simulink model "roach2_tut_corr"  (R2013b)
settings: Solver=VariableStepDiscrete  SolverMode=SingleTasking  StartTime=0.0  StopTime=100  RelTol=1e-3
undefined symbols (not defined in the file): add_latency, addr_width, Bit, bitfield, BitWidth, bram_latency, burst_size, casper_library_scopes, conv_latency, data_width, DelayLen, fan_latency, FFTSize, FFTStage, getfield, increment, led, Location, Lower, mult_latency, mux_latency, n_bits, n_bits_data, n_inputs, n_streams, n_taps, neg_latency, negate_latency, nsamples, pfb_size, pulse_len, reset_period, ROACH, ROACH2, snapshot, sx475t, sync_period, sync_period_bits, Upper, UseCounter, Width
libraries: xbsIndex_r4 x24444, casper_library_misc x73, xbsReplacements_r4 x34, casper_library_delays x14, xps_library x7
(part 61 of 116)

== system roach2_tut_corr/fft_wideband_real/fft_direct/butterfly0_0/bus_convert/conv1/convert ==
  note: (ones_bit & 1) -> round-to-even (ones_bit ^ 1) -> round-to-odd (sign_bit & 1)-> round-to-zero (sign_bit ^ 1) -> round-to-inf (X ~| 1) -> round half down (X | 1) -> round half up
  in : Inport
  Concat : xbsIndex_r4/Concat  num_inputs=2  dbl_ovrd=off  block_type=concat
  Constant : xbsIndex_r4/Constant  const=1  gui_display_data_type=Fixed-point  arith_type=Unsigned  n_bits=1  bin_pt=0  preci_type=Single  exp_width=8  frac_width=24  explicit_period=off  period=1  equ=P=C  opselect=C  inp2=PCIN>>17  opr=+  inp1=P  carry=CIN  dbl_ovrd=off  block_type=constant
  Reinterpret : xbsIndex_r4/Reinterpret  force_arith_type=on  arith_type=Unsigned  force_bin_pt=on  bin_pt=0  block_type=reinterpret
  adder : xbsIndex_r4/AddSub  mode=Addition  use_carryin=off  use_carryout=off  en=off  latency=1  precision=User Defined  arith_type="Signed  (2's comp)"  n_bits=18  bin_pt=17  quantization=Truncate  overflow=Wrap  dbl_ovrd=off  use_behavioral_HDL=off  hw_selection=Fabric  pipelined=on  use_rpm=on  block_type=addsub
  almost_half : xbsIndex_r4/Constant  const=1  gui_display_data_type=Fixed-point  arith_type=Unsigned  n_bits=19  bin_pt=0  preci_type=Single  exp_width=8  frac_width=24  explicit_period=off  period=1  equ=P=C  opselect=C  inp2=PCIN>>17  opr=+  inp1=P  carry=CIN  dbl_ovrd=off  block_type=constant
  bit : xbsIndex_r4/Slice  nbits=1  boolean_output=off  mode=Lower Bit Location + Width  bit1=0  base1=MSB of Input  bit0=1  base0=LSB of Input  dbl_ovrd=off  block_type=slice
  force1 : xbsIndex_r4/Reinterpret  force_arith_type=on  arith_type="Signed  (2's comp)"  force_bin_pt=on  bin_pt=19  block_type=reinterpret
  force2 : xbsIndex_r4/Reinterpret  force_arith_type=off  arith_type="Signed  (2's comp)"  force_bin_pt=on  bin_pt=19  block_type=reinterpret
  tweak_op : xbsIndex_r4/Logical  logical_function=AND  inputs=2  en=off  latency=0  precision=Full  arith_type=Unsigned  n_bits=8  bin_pt=2  align_bp=on  dbl_ovrd=off  block_type=logical
  out : Outport
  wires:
  tweak_op/1 -> Concat/2
  Constant/1 -> tweak_op/2
  bit/1 -> tweak_op/1
  almost_half/1 -> force2/1
  in/1 -> Reinterpret/1, bit/1
  Concat/1 -> force1/1
  Reinterpret/1 -> Concat/1
  force1/1 -> adder/1
  force2/1 -> adder/2
  adder/1 -> out/1

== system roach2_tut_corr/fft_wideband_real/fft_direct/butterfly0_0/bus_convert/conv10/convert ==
  note: (ones_bit & 1) -> round-to-even (ones_bit ^ 1) -> round-to-odd (sign_bit & 1)-> round-to-zero (sign_bit ^ 1) -> round-to-inf (X ~| 1) -> round half down (X | 1) -> round half up
  in : Inport
  Concat : xbsIndex_r4/Concat  num_inputs=2  dbl_ovrd=off  block_type=concat
  Constant : xbsIndex_r4/Constant  const=1  gui_display_data_type=Fixed-point  arith_type=Unsigned  n_bits=1  bin_pt=0  preci_type=Single  exp_width=8  frac_width=24  explicit_period=off  period=1  equ=P=C  opselect=C  inp2=PCIN>>17  opr=+  inp1=P  carry=CIN  dbl_ovrd=off  block_type=constant
  Reinterpret : xbsIndex_r4/Reinterpret  force_arith_type=on  arith_type=Unsigned  force_bin_pt=on  bin_pt=0  block_type=reinterpret
  adder : xbsIndex_r4/AddSub  mode=Addition  use_carryin=off  use_carryout=off  en=off  latency=1  precision=User Defined  arith_type="Signed  (2's comp)"  n_bits=18  bin_pt=17  quantization=Truncate  overflow=Wrap  dbl_ovrd=off  use_behavioral_HDL=off  hw_selection=Fabric  pipelined=on  use_rpm=on  block_type=addsub
  almost_half : xbsIndex_r4/Constant  const=1  gui_display_data_type=Fixed-point  arith_type=Unsigned  n_bits=19  bin_pt=0  preci_type=Single  exp_width=8  frac_width=24  explicit_period=off  period=1  equ=P=C  opselect=C  inp2=PCIN>>17  opr=+  inp1=P  carry=CIN  dbl_ovrd=off  block_type=constant
  bit : xbsIndex_r4/Slice  nbits=1  boolean_output=off  mode=Lower Bit Location + Width  bit1=0  base1=MSB of Input  bit0=1  base0=LSB of Input  dbl_ovrd=off  block_type=slice
  force1 : xbsIndex_r4/Reinterpret  force_arith_type=on  arith_type="Signed  (2's comp)"  force_bin_pt=on  bin_pt=19  block_type=reinterpret
  force2 : xbsIndex_r4/Reinterpret  force_arith_type=off  arith_type="Signed  (2's comp)"  force_bin_pt=on  bin_pt=19  block_type=reinterpret
  tweak_op : xbsIndex_r4/Logical  logical_function=AND  inputs=2  en=off  latency=0  precision=Full  arith_type=Unsigned  n_bits=8  bin_pt=2  align_bp=on  dbl_ovrd=off  block_type=logical
  out : Outport
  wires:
  tweak_op/1 -> Concat/2
  Constant/1 -> tweak_op/2
  bit/1 -> tweak_op/1
  almost_half/1 -> force2/1
  in/1 -> Reinterpret/1, bit/1
  Concat/1 -> force1/1
  Reinterpret/1 -> Concat/1
  force1/1 -> adder/1
  force2/1 -> adder/2
  adder/1 -> out/1

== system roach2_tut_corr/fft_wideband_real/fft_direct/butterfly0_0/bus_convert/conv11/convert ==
  note: (ones_bit & 1) -> round-to-even (ones_bit ^ 1) -> round-to-odd (sign_bit & 1)-> round-to-zero (sign_bit ^ 1) -> round-to-inf (X ~| 1) -> round half down (X | 1) -> round half up
  in : Inport
  Concat : xbsIndex_r4/Concat  num_inputs=2  dbl_ovrd=off  block_type=concat
  Constant : xbsIndex_r4/Constant  const=1  gui_display_data_type=Fixed-point  arith_type=Unsigned  n_bits=1  bin_pt=0  preci_type=Single  exp_width=8  frac_width=24  explicit_period=off  period=1  equ=P=C  opselect=C  inp2=PCIN>>17  opr=+  inp1=P  carry=CIN  dbl_ovrd=off  block_type=constant
  Reinterpret : xbsIndex_r4/Reinterpret  force_arith_type=on  arith_type=Unsigned  force_bin_pt=on  bin_pt=0  block_type=reinterpret
  adder : xbsIndex_r4/AddSub  mode=Addition  use_carryin=off  use_carryout=off  en=off  latency=1  precision=User Defined  arith_type="Signed  (2's comp)"  n_bits=18  bin_pt=17  quantization=Truncate  overflow=Wrap  dbl_ovrd=off  use_behavioral_HDL=off  hw_selection=Fabric  pipelined=on  use_rpm=on  block_type=addsub
  almost_half : xbsIndex_r4/Constant  const=1  gui_display_data_type=Fixed-point  arith_type=Unsigned  n_bits=19  bin_pt=0  preci_type=Single  exp_width=8  frac_width=24  explicit_period=off  period=1  equ=P=C  opselect=C  inp2=PCIN>>17  opr=+  inp1=P  carry=CIN  dbl_ovrd=off  block_type=constant
  bit : xbsIndex_r4/Slice  nbits=1  boolean_output=off  mode=Lower Bit Location + Width  bit1=0  base1=MSB of Input  bit0=1  base0=LSB of Input  dbl_ovrd=off  block_type=slice
  force1 : xbsIndex_r4/Reinterpret  force_arith_type=on  arith_type="Signed  (2's comp)"  force_bin_pt=on  bin_pt=19  block_type=reinterpret
  force2 : xbsIndex_r4/Reinterpret  force_arith_type=off  arith_type="Signed  (2's comp)"  force_bin_pt=on  bin_pt=19  block_type=reinterpret
  tweak_op : xbsIndex_r4/Logical  logical_function=AND  inputs=2  en=off  latency=0  precision=Full  arith_type=Unsigned  n_bits=8  bin_pt=2  align_bp=on  dbl_ovrd=off  block_type=logical
  out : Outport
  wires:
  tweak_op/1 -> Concat/2
  Constant/1 -> tweak_op/2
  bit/1 -> tweak_op/1
  almost_half/1 -> force2/1
  in/1 -> Reinterpret/1, bit/1
  Concat/1 -> force1/1
  Reinterpret/1 -> Concat/1
  force1/1 -> adder/1
  force2/1 -> adder/2
  adder/1 -> out/1

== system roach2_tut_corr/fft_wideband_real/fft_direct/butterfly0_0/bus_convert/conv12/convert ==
  note: (ones_bit & 1) -> round-to-even (ones_bit ^ 1) -> round-to-odd (sign_bit & 1)-> round-to-zero (sign_bit ^ 1) -> round-to-inf (X ~| 1) -> round half down (X | 1) -> round half up
  in : Inport
  Concat : xbsIndex_r4/Concat  num_inputs=2  dbl_ovrd=off  block_type=concat
  Constant : xbsIndex_r4/Constant  const=1  gui_display_data_type=Fixed-point  arith_type=Unsigned  n_bits=1  bin_pt=0  preci_type=Single  exp_width=8  frac_width=24  explicit_period=off  period=1  equ=P=C  opselect=C  inp2=PCIN>>17  opr=+  inp1=P  carry=CIN  dbl_ovrd=off  block_type=constant
  Reinterpret : xbsIndex_r4/Reinterpret  force_arith_type=on  arith_type=Unsigned  force_bin_pt=on  bin_pt=0  block_type=reinterpret
  adder : xbsIndex_r4/AddSub  mode=Addition  use_carryin=off  use_carryout=off  en=off  latency=1  precision=User Defined  arith_type="Signed  (2's comp)"  n_bits=18  bin_pt=17  quantization=Truncate  overflow=Wrap  dbl_ovrd=off  use_behavioral_HDL=off  hw_selection=Fabric  pipelined=on  use_rpm=on  block_type=addsub
  almost_half : xbsIndex_r4/Constant  const=1  gui_display_data_type=Fixed-point  arith_type=Unsigned  n_bits=19  bin_pt=0  preci_type=Single  exp_width=8  frac_width=24  explicit_period=off  period=1  equ=P=C  opselect=C  inp2=PCIN>>17  opr=+  inp1=P  carry=CIN  dbl_ovrd=off  block_type=constant
  bit : xbsIndex_r4/Slice  nbits=1  boolean_output=off  mode=Lower Bit Location + Width  bit1=0  base1=MSB of Input  bit0=1  base0=LSB of Input  dbl_ovrd=off  block_type=slice
  force1 : xbsIndex_r4/Reinterpret  force_arith_type=on  arith_type="Signed  (2's comp)"  force_bin_pt=on  bin_pt=19  block_type=reinterpret
  force2 : xbsIndex_r4/Reinterpret  force_arith_type=off  arith_type="Signed  (2's comp)"  force_bin_pt=on  bin_pt=19  block_type=reinterpret
  tweak_op : xbsIndex_r4/Logical  logical_function=AND  inputs=2  en=off  latency=0  precision=Full  arith_type=Unsigned  n_bits=8  bin_pt=2  align_bp=on  dbl_ovrd=off  block_type=logical
  out : Outport
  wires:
  tweak_op/1 -> Concat/2
  Constant/1 -> tweak_op/2
  bit/1 -> tweak_op/1
  almost_half/1 -> force2/1
  in/1 -> Reinterpret/1, bit/1
  Concat/1 -> force1/1
  Reinterpret/1 -> Concat/1
  force1/1 -> adder/1
  force2/1 -> adder/2
  adder/1 -> out/1

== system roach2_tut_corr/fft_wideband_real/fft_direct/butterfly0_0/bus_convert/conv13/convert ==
  note: (ones_bit & 1) -> round-to-even (ones_bit ^ 1) -> round-to-odd (sign_bit & 1)-> round-to-zero (sign_bit ^ 1) -> round-to-inf (X ~| 1) -> round half down (X | 1) -> round half up
  in : Inport
  Concat : xbsIndex_r4/Concat  num_inputs=2  dbl_ovrd=off  block_type=concat
  Constant : xbsIndex_r4/Constant  const=1  gui_display_data_type=Fixed-point  arith_type=Unsigned  n_bits=1  bin_pt=0  preci_type=Single  exp_width=8  frac_width=24  explicit_period=off  period=1  equ=P=C  opselect=C  inp2=PCIN>>17  opr=+  inp1=P  carry=CIN  dbl_ovrd=off  block_type=constant
  Reinterpret : xbsIndex_r4/Reinterpret  force_arith_type=on  arith_type=Unsigned  force_bin_pt=on  bin_pt=0  block_type=reinterpret
  adder : xbsIndex_r4/AddSub  mode=Addition  use_carryin=off  use_carryout=off  en=off  latency=1  precision=User Defined  arith_type="Signed  (2's comp)"  n_bits=18  bin_pt=17  quantization=Truncate  overflow=Wrap  dbl_ovrd=off  use_behavioral_HDL=off  hw_selection=Fabric  pipelined=on  use_rpm=on  block_type=addsub
  almost_half : xbsIndex_r4/Constant  const=1  gui_display_data_type=Fixed-point  arith_type=Unsigned  n_bits=19  bin_pt=0  preci_type=Single  exp_width=8  frac_width=24  explicit_period=off  period=1  equ=P=C  opselect=C  inp2=PCIN>>17  opr=+  inp1=P  carry=CIN  dbl_ovrd=off  block_type=constant
  bit : xbsIndex_r4/Slice  nbits=1  boolean_output=off  mode=Lower Bit Location + Width  bit1=0  base1=MSB of Input  bit0=1  base0=LSB of Input  dbl_ovrd=off  block_type=slice
  force1 : xbsIndex_r4/Reinterpret  force_arith_type=on  arith_type="Signed  (2's comp)"  force_bin_pt=on  bin_pt=19  block_type=reinterpret
  force2 : xbsIndex_r4/Reinterpret  force_arith_type=off  arith_type="Signed  (2's comp)"  force_bin_pt=on  bin_pt=19  block_type=reinterpret
  tweak_op : xbsIndex_r4/Logical  logical_function=AND  inputs=2  en=off  latency=0  precision=Full  arith_type=Unsigned  n_bits=8  bin_pt=2  align_bp=on  dbl_ovrd=off  block_type=logical
  out : Outport
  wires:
  tweak_op/1 -> Concat/2
  Constant/1 -> tweak_op/2
  bit/1 -> tweak_op/1
  almost_half/1 -> force2/1
  in/1 -> Reinterpret/1, bit/1
  Concat/1 -> force1/1
  Reinterpret/1 -> Concat/1
  force1/1 -> adder/1
  force2/1 -> adder/2
  adder/1 -> out/1

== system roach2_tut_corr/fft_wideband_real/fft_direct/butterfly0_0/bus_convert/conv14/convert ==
  note: (ones_bit & 1) -> round-to-even (ones_bit ^ 1) -> round-to-odd (sign_bit & 1)-> round-to-zero (sign_bit ^ 1) -> round-to-inf (X ~| 1) -> round half down (X | 1) -> round half up
  in : Inport
  Concat : xbsIndex_r4/Concat  num_inputs=2  dbl_ovrd=off  block_type=concat
  Constant : xbsIndex_r4/Constant  const=1  gui_display_data_type=Fixed-point  arith_type=Unsigned  n_bits=1  bin_pt=0  preci_type=Single  exp_width=8  frac_width=24  explicit_period=off  period=1  equ=P=C  opselect=C  inp2=PCIN>>17  opr=+  inp1=P  carry=CIN  dbl_ovrd=off  block_type=constant
  Reinterpret : xbsIndex_r4/Reinterpret  force_arith_type=on  arith_type=Unsigned  force_bin_pt=on  bin_pt=0  block_type=reinterpret
  adder : xbsIndex_r4/AddSub  mode=Addition  use_carryin=off  use_carryout=off  en=off  latency=1  precision=User Defined  arith_type="Signed  (2's comp)"  n_bits=18  bin_pt=17  quantization=Truncate  overflow=Wrap  dbl_ovrd=off  use_behavioral_HDL=off  hw_selection=Fabric  pipelined=on  use_rpm=on  block_type=addsub
  almost_half : xbsIndex_r4/Constant  const=1  gui_display_data_type=Fixed-point  arith_type=Unsigned  n_bits=19  bin_pt=0  preci_type=Single  exp_width=8  frac_width=24  explicit_period=off  period=1  equ=P=C  opselect=C  inp2=PCIN>>17  opr=+  inp1=P  carry=CIN  dbl_ovrd=off  block_type=constant
  bit : xbsIndex_r4/Slice  nbits=1  boolean_output=off  mode=Lower Bit Location + Width  bit1=0  base1=MSB of Input  bit0=1  base0=LSB of Input  dbl_ovrd=off  block_type=slice
  force1 : xbsIndex_r4/Reinterpret  force_arith_type=on  arith_type="Signed  (2's comp)"  force_bin_pt=on  bin_pt=19  block_type=reinterpret
  force2 : xbsIndex_r4/Reinterpret  force_arith_type=off  arith_type="Signed  (2's comp)"  force_bin_pt=on  bin_pt=19  block_type=reinterpret
  tweak_op : xbsIndex_r4/Logical  logical_function=AND  inputs=2  en=off  latency=0  precision=Full  arith_type=Unsigned  n_bits=8  bin_pt=2  align_bp=on  dbl_ovrd=off  block_type=logical
  out : Outport
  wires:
  tweak_op/1 -> Concat/2
  Constant/1 -> tweak_op/2
  bit/1 -> tweak_op/1
  almost_half/1 -> force2/1
  in/1 -> Reinterpret/1, bit/1
  Concat/1 -> force1/1
  Reinterpret/1 -> Concat/1
  force1/1 -> adder/1
  force2/1 -> adder/2
  adder/1 -> out/1

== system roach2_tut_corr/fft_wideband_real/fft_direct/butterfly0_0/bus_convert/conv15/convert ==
  note: (ones_bit & 1) -> round-to-even (ones_bit ^ 1) -> round-to-odd (sign_bit & 1)-> round-to-zero (sign_bit ^ 1) -> round-to-inf (X ~| 1) -> round half down (X | 1) -> round half up
  in : Inport
  Concat : xbsIndex_r4/Concat  num_inputs=2  dbl_ovrd=off  block_type=concat
  Constant : xbsIndex_r4/Constant  const=1  gui_display_data_type=Fixed-point  arith_type=Unsigned  n_bits=1  bin_pt=0  preci_type=Single  exp_width=8  frac_width=24  explicit_period=off  period=1  equ=P=C  opselect=C  inp2=PCIN>>17  opr=+  inp1=P  carry=CIN  dbl_ovrd=off  block_type=constant
  Reinterpret : xbsIndex_r4/Reinterpret  force_arith_type=on  arith_type=Unsigned  force_bin_pt=on  bin_pt=0  block_type=reinterpret
  adder : xbsIndex_r4/AddSub  mode=Addition  use_carryin=off  use_carryout=off  en=off  latency=1  precision=User Defined  arith_type="Signed  (2's comp)"  n_bits=18  bin_pt=17  quantization=Truncate  overflow=Wrap  dbl_ovrd=off  use_behavioral_HDL=off  hw_selection=Fabric  pipelined=on  use_rpm=on  block_type=addsub
  almost_half : xbsIndex_r4/Constant  const=1  gui_display_data_type=Fixed-point  arith_type=Unsigned  n_bits=19  bin_pt=0  preci_type=Single  exp_width=8  frac_width=24  explicit_period=off  period=1  equ=P=C  opselect=C  inp2=PCIN>>17  opr=+  inp1=P  carry=CIN  dbl_ovrd=off  block_type=constant
  bit : xbsIndex_r4/Slice  nbits=1  boolean_output=off  mode=Lower Bit Location + Width  bit1=0  base1=MSB of Input  bit0=1  base0=LSB of Input  dbl_ovrd=off  block_type=slice
  force1 : xbsIndex_r4/Reinterpret  force_arith_type=on  arith_type="Signed  (2's comp)"  force_bin_pt=on  bin_pt=19  block_type=reinterpret
  force2 : xbsIndex_r4/Reinterpret  force_arith_type=off  arith_type="Signed  (2's comp)"  force_bin_pt=on  bin_pt=19  block_type=reinterpret
  tweak_op : xbsIndex_r4/Logical  logical_function=AND  inputs=2  en=off  latency=0  precision=Full  arith_type=Unsigned  n_bits=8  bin_pt=2  align_bp=on  dbl_ovrd=off  block_type=logical
  out : Outport
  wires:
  tweak_op/1 -> Concat/2
  Constant/1 -> tweak_op/2
  bit/1 -> tweak_op/1
  almost_half/1 -> force2/1
  in/1 -> Reinterpret/1, bit/1
  Concat/1 -> force1/1
  Reinterpret/1 -> Concat/1
  force1/1 -> adder/1
  force2/1 -> adder/2
  adder/1 -> out/1

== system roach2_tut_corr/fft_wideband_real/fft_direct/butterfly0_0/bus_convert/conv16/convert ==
  note: (ones_bit & 1) -> round-to-even (ones_bit ^ 1) -> round-to-odd (sign_bit & 1)-> round-to-zero (sign_bit ^ 1) -> round-to-inf (X ~| 1) -> round half down (X | 1) -> round half up
  in : Inport
  Concat : xbsIndex_r4/Concat  num_inputs=2  dbl_ovrd=off  block_type=concat
  Constant : xbsIndex_r4/Constant  const=1  gui_display_data_type=Fixed-point  arith_type=Unsigned  n_bits=1  bin_pt=0  preci_type=Single  exp_width=8  frac_width=24  explicit_period=off  period=1  equ=P=C  opselect=C  inp2=PCIN>>17  opr=+  inp1=P  carry=CIN  dbl_ovrd=off  block_type=constant
  Reinterpret : xbsIndex_r4/Reinterpret  force_arith_type=on  arith_type=Unsigned  force_bin_pt=on  bin_pt=0  block_type=reinterpret
  adder : xbsIndex_r4/AddSub  mode=Addition  use_carryin=off  use_carryout=off  en=off  latency=1  precision=User Defined  arith_type="Signed  (2's comp)"  n_bits=18  bin_pt=17  quantization=Truncate  overflow=Wrap  dbl_ovrd=off  use_behavioral_HDL=off  hw_selection=Fabric  pipelined=on  use_rpm=on  block_type=addsub
  almost_half : xbsIndex_r4/Constant  const=1  gui_display_data_type=Fixed-point  arith_type=Unsigned  n_bits=19  bin_pt=0  preci_type=Single  exp_width=8  frac_width=24  explicit_period=off  period=1  equ=P=C  opselect=C  inp2=PCIN>>17  opr=+  inp1=P  carry=CIN  dbl_ovrd=off  block_type=constant
  bit : xbsIndex_r4/Slice  nbits=1  boolean_output=off  mode=Lower Bit Location + Width  bit1=0  base1=MSB of Input  bit0=1  base0=LSB of Input  dbl_ovrd=off  block_type=slice
  force1 : xbsIndex_r4/Reinterpret  force_arith_type=on  arith_type="Signed  (2's comp)"  force_bin_pt=on  bin_pt=19  block_type=reinterpret
  force2 : xbsIndex_r4/Reinterpret  force_arith_type=off  arith_type="Signed  (2's comp)"  force_bin_pt=on  bin_pt=19  block_type=reinterpret
  tweak_op : xbsIndex_r4/Logical  logical_function=AND  inputs=2  en=off  latency=0  precision=Full  arith_type=Unsigned  n_bits=8  bin_pt=2  align_bp=on  dbl_ovrd=off  block_type=logical
  out : Outport
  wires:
  tweak_op/1 -> Concat/2
  Constant/1 -> tweak_op/2
  bit/1 -> tweak_op/1
  almost_half/1 -> force2/1
  in/1 -> Reinterpret/1, bit/1
  Concat/1 -> force1/1
  Reinterpret/1 -> Concat/1
  force1/1 -> adder/1
  force2/1 -> adder/2
  adder/1 -> out/1

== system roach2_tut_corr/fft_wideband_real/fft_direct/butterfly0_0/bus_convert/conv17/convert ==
  note: (ones_bit & 1) -> round-to-even (ones_bit ^ 1) -> round-to-odd (sign_bit & 1)-> round-to-zero (sign_bit ^ 1) -> round-to-inf (X ~| 1) -> round half down (X | 1) -> round half up
  in : Inport
  Concat : xbsIndex_r4/Concat  num_inputs=2  dbl_ovrd=off  block_type=concat
  Constant : xbsIndex_r4/Constant  const=1  gui_display_data_type=Fixed-point  arith_type=Unsigned  n_bits=1  bin_pt=0  preci_type=Single  exp_width=8  frac_width=24  explicit_period=off  period=1  equ=P=C  opselect=C  inp2=PCIN>>17  opr=+  inp1=P  carry=CIN  dbl_ovrd=off  block_type=constant
  Reinterpret : xbsIndex_r4/Reinterpret  force_arith_type=on  arith_type=Unsigned  force_bin_pt=on  bin_pt=0  block_type=reinterpret
  adder : xbsIndex_r4/AddSub  mode=Addition  use_carryin=off  use_carryout=off  en=off  latency=1  precision=User Defined  arith_type="Signed  (2's comp)"  n_bits=18  bin_pt=17  quantization=Truncate  overflow=Wrap  dbl_ovrd=off  use_behavioral_HDL=off  hw_selection=Fabric  pipelined=on  use_rpm=on  block_type=addsub
  almost_half : xbsIndex_r4/Constant  const=1  gui_display_data_type=Fixed-point  arith_type=Unsigned  n_bits=19  bin_pt=0  preci_type=Single  exp_width=8  frac_width=24  explicit_period=off  period=1  equ=P=C  opselect=C  inp2=PCIN>>17  opr=+  inp1=P  carry=CIN  dbl_ovrd=off  block_type=constant
  bit : xbsIndex_r4/Slice  nbits=1  boolean_output=off  mode=Lower Bit Location + Width  bit1=0  base1=MSB of Input  bit0=1  base0=LSB of Input  dbl_ovrd=off  block_type=slice
  force1 : xbsIndex_r4/Reinterpret  force_arith_type=on  arith_type="Signed  (2's comp)"  force_bin_pt=on  bin_pt=19  block_type=reinterpret
  force2 : xbsIndex_r4/Reinterpret  force_arith_type=off  arith_type="Signed  (2's comp)"  force_bin_pt=on  bin_pt=19  block_type=reinterpret
  tweak_op : xbsIndex_r4/Logical  logical_function=AND  inputs=2  en=off  latency=0  precision=Full  arith_type=Unsigned  n_bits=8  bin_pt=2  align_bp=on  dbl_ovrd=off  block_type=logical
  out : Outport
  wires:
  tweak_op/1 -> Concat/2
  Constant/1 -> tweak_op/2
  bit/1 -> tweak_op/1
  almost_half/1 -> force2/1
  in/1 -> Reinterpret/1, bit/1
  Concat/1 -> force1/1
  Reinterpret/1 -> Concat/1
  force1/1 -> adder/1
  force2/1 -> adder/2
  adder/1 -> out/1

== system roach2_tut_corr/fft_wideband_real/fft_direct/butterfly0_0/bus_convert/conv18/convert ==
  note: (ones_bit & 1) -> round-to-even (ones_bit ^ 1) -> round-to-odd (sign_bit & 1)-> round-to-zero (sign_bit ^ 1) -> round-to-inf (X ~| 1) -> round half down (X | 1) -> round half up
  in : Inport
  Concat : xbsIndex_r4/Concat  num_inputs=2  dbl_ovrd=off  block_type=concat
  Constant : xbsIndex_r4/Constant  const=1  gui_display_data_type=Fixed-point  arith_type=Unsigned  n_bits=1  bin_pt=0  preci_type=Single  exp_width=8  frac_width=24  explicit_period=off  period=1  equ=P=C  opselect=C  inp2=PCIN>>17  opr=+  inp1=P  carry=CIN  dbl_ovrd=off  block_type=constant
  Reinterpret : xbsIndex_r4/Reinterpret  force_arith_type=on  arith_type=Unsigned  force_bin_pt=on  bin_pt=0  block_type=reinterpret
  adder : xbsIndex_r4/AddSub  mode=Addition  use_carryin=off  use_carryout=off  en=off  latency=1  precision=User Defined  arith_type="Signed  (2's comp)"  n_bits=18  bin_pt=17  quantization=Truncate  overflow=Wrap  dbl_ovrd=off  use_behavioral_HDL=off  hw_selection=Fabric  pipelined=on  use_rpm=on  block_type=addsub
  almost_half : xbsIndex_r4/Constant  const=1  gui_display_data_type=Fixed-point  arith_type=Unsigned  n_bits=19  bin_pt=0  preci_type=Single  exp_width=8  frac_width=24  explicit_period=off  period=1  equ=P=C  opselect=C  inp2=PCIN>>17  opr=+  inp1=P  carry=CIN  dbl_ovrd=off  block_type=constant
  bit : xbsIndex_r4/Slice  nbits=1  boolean_output=off  mode=Lower Bit Location + Width  bit1=0  base1=MSB of Input  bit0=1  base0=LSB of Input  dbl_ovrd=off  block_type=slice
  force1 : xbsIndex_r4/Reinterpret  force_arith_type=on  arith_type="Signed  (2's comp)"  force_bin_pt=on  bin_pt=19  block_type=reinterpret
  force2 : xbsIndex_r4/Reinterpret  force_arith_type=off  arith_type="Signed  (2's comp)"  force_bin_pt=on  bin_pt=19  block_type=reinterpret
  tweak_op : xbsIndex_r4/Logical  logical_function=AND  inputs=2  en=off  latency=0  precision=Full  arith_type=Unsigned  n_bits=8  bin_pt=2  align_bp=on  dbl_ovrd=off  block_type=logical
  out : Outport
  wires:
  tweak_op/1 -> Concat/2
  Constant/1 -> tweak_op/2
  bit/1 -> tweak_op/1
  almost_half/1 -> force2/1
  in/1 -> Reinterpret/1, bit/1
  Concat/1 -> force1/1
  Reinterpret/1 -> Concat/1
  force1/1 -> adder/1
  force2/1 -> adder/2
  adder/1 -> out/1

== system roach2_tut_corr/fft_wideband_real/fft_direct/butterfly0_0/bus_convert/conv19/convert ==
  note: (ones_bit & 1) -> round-to-even (ones_bit ^ 1) -> round-to-odd (sign_bit & 1)-> round-to-zero (sign_bit ^ 1) -> round-to-inf (X ~| 1) -> round half down (X | 1) -> round half up
  in : Inport
  Concat : xbsIndex_r4/Concat  num_inputs=2  dbl_ovrd=off  block_type=concat
  Constant : xbsIndex_r4/Constant  const=1  gui_display_data_type=Fixed-point  arith_type=Unsigned  n_bits=1  bin_pt=0  preci_type=Single  exp_width=8  frac_width=24  explicit_period=off  period=1  equ=P=C  opselect=C  inp2=PCIN>>17  opr=+  inp1=P  carry=CIN  dbl_ovrd=off  block_type=constant
  Reinterpret : xbsIndex_r4/Reinterpret  force_arith_type=on  arith_type=Unsigned  force_bin_pt=on  bin_pt=0  block_type=reinterpret
  adder : xbsIndex_r4/AddSub  mode=Addition  use_carryin=off  use_carryout=off  en=off  latency=1  precision=User Defined  arith_type="Signed  (2's comp)"  n_bits=18  bin_pt=17  quantization=Truncate  overflow=Wrap  dbl_ovrd=off  use_behavioral_HDL=off  hw_selection=Fabric  pipelined=on  use_rpm=on  block_type=addsub
  almost_half : xbsIndex_r4/Constant  const=1  gui_display_data_type=Fixed-point  arith_type=Unsigned  n_bits=19  bin_pt=0  preci_type=Single  exp_width=8  frac_width=24  explicit_period=off  period=1  equ=P=C  opselect=C  inp2=PCIN>>17  opr=+  inp1=P  carry=CIN  dbl_ovrd=off  block_type=constant
  bit : xbsIndex_r4/Slice  nbits=1  boolean_output=off  mode=Lower Bit Location + Width  bit1=0  base1=MSB of Input  bit0=1  base0=LSB of Input  dbl_ovrd=off  block_type=slice
  force1 : xbsIndex_r4/Reinterpret  force_arith_type=on  arith_type="Signed  (2's comp)"  force_bin_pt=on  bin_pt=19  block_type=reinterpret
  force2 : xbsIndex_r4/Reinterpret  force_arith_type=off  arith_type="Signed  (2's comp)"  force_bin_pt=on  bin_pt=19  block_type=reinterpret
  tweak_op : xbsIndex_r4/Logical  logical_function=AND  inputs=2  en=off  latency=0  precision=Full  arith_type=Unsigned  n_bits=8  bin_pt=2  align_bp=on  dbl_ovrd=off  block_type=logical
  out : Outport
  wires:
  tweak_op/1 -> Concat/2
  Constant/1 -> tweak_op/2
  bit/1 -> tweak_op/1
  almost_half/1 -> force2/1
  in/1 -> Reinterpret/1, bit/1
  Concat/1 -> force1/1
  Reinterpret/1 -> Concat/1
  force1/1 -> adder/1
  force2/1 -> adder/2
  adder/1 -> out/1

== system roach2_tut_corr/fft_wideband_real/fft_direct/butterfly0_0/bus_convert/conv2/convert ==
  note: (ones_bit & 1) -> round-to-even (ones_bit ^ 1) -> round-to-odd (sign_bit & 1)-> round-to-zero (sign_bit ^ 1) -> round-to-inf (X ~| 1) -> round half down (X | 1) -> round half up
  in : Inport
  Concat : xbsIndex_r4/Concat  num_inputs=2  dbl_ovrd=off  block_type=concat
  Constant : xbsIndex_r4/Constant  const=1  gui_display_data_type=Fixed-point  arith_type=Unsigned  n_bits=1  bin_pt=0  preci_type=Single  exp_width=8  frac_width=24  explicit_period=off  period=1  equ=P=C  opselect=C  inp2=PCIN>>17  opr=+  inp1=P  carry=CIN  dbl_ovrd=off  block_type=constant
  Reinterpret : xbsIndex_r4/Reinterpret  force_arith_type=on  arith_type=Unsigned  force_bin_pt=on  bin_pt=0  block_type=reinterpret
  adder : xbsIndex_r4/AddSub  mode=Addition  use_carryin=off  use_carryout=off  en=off  latency=1  precision=User Defined  arith_type="Signed  (2's comp)"  n_bits=18  bin_pt=17  quantization=Truncate  overflow=Wrap  dbl_ovrd=off  use_behavioral_HDL=off  hw_selection=Fabric  pipelined=on  use_rpm=on  block_type=addsub
  almost_half : xbsIndex_r4/Constant  const=1  gui_display_data_type=Fixed-point  arith_type=Unsigned  n_bits=19  bin_pt=0  preci_type=Single  exp_width=8  frac_width=24  explicit_period=off  period=1  equ=P=C  opselect=C  inp2=PCIN>>17  opr=+  inp1=P  carry=CIN  dbl_ovrd=off  block_type=constant
  bit : xbsIndex_r4/Slice  nbits=1  boolean_output=off  mode=Lower Bit Location + Width  bit1=0  base1=MSB of Input  bit0=1  base0=LSB of Input  dbl_ovrd=off  block_type=slice
  force1 : xbsIndex_r4/Reinterpret  force_arith_type=on  arith_type="Signed  (2's comp)"  force_bin_pt=on  bin_pt=19  block_type=reinterpret
  force2 : xbsIndex_r4/Reinterpret  force_arith_type=off  arith_type="Signed  (2's comp)"  force_bin_pt=on  bin_pt=19  block_type=reinterpret
  tweak_op : xbsIndex_r4/Logical  logical_function=AND  inputs=2  en=off  latency=0  precision=Full  arith_type=Unsigned  n_bits=8  bin_pt=2  align_bp=on  dbl_ovrd=off  block_type=logical
  out : Outport
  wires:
  tweak_op/1 -> Concat/2
  Constant/1 -> tweak_op/2
  bit/1 -> tweak_op/1
  almost_half/1 -> force2/1
  in/1 -> Reinterpret/1, bit/1
  Concat/1 -> force1/1
  Reinterpret/1 -> Concat/1
  force1/1 -> adder/1
  force2/1 -> adder/2
  adder/1 -> out/1

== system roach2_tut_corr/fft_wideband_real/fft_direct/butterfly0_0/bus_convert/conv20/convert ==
  note: (ones_bit & 1) -> round-to-even (ones_bit ^ 1) -> round-to-odd (sign_bit & 1)-> round-to-zero (sign_bit ^ 1) -> round-to-inf (X ~| 1) -> round half down (X | 1) -> round half up
  in : Inport
  Concat : xbsIndex_r4/Concat  num_inputs=2  dbl_ovrd=off  block_type=concat
  Constant : xbsIndex_r4/Constant  const=1  gui_display_data_type=Fixed-point  arith_type=Unsigned  n_bits=1  bin_pt=0  preci_type=Single  exp_width=8  frac_width=24  explicit_period=off  period=1  equ=P=C  opselect=C  inp2=PCIN>>17  opr=+  inp1=P  carry=CIN  dbl_ovrd=off  block_type=constant
  Reinterpret : xbsIndex_r4/Reinterpret  force_arith_type=on  arith_type=Unsigned  force_bin_pt=on  bin_pt=0  block_type=reinterpret
  adder : xbsIndex_r4/AddSub  mode=Addition  use_carryin=off  use_carryout=off  en=off  latency=1  precision=User Defined  arith_type="Signed  (2's comp)"  n_bits=18  bin_pt=17  quantization=Truncate  overflow=Wrap  dbl_ovrd=off  use_behavioral_HDL=off  hw_selection=Fabric  pipelined=on  use_rpm=on  block_type=addsub
  almost_half : xbsIndex_r4/Constant  const=1  gui_display_data_type=Fixed-point  arith_type=Unsigned  n_bits=19  bin_pt=0  preci_type=Single  exp_width=8  frac_width=24  explicit_period=off  period=1  equ=P=C  opselect=C  inp2=PCIN>>17  opr=+  inp1=P  carry=CIN  dbl_ovrd=off  block_type=constant
  bit : xbsIndex_r4/Slice  nbits=1  boolean_output=off  mode=Lower Bit Location + Width  bit1=0  base1=MSB of Input  bit0=1  base0=LSB of Input  dbl_ovrd=off  block_type=slice
  force1 : xbsIndex_r4/Reinterpret  force_arith_type=on  arith_type="Signed  (2's comp)"  force_bin_pt=on  bin_pt=19  block_type=reinterpret
  force2 : xbsIndex_r4/Reinterpret  force_arith_type=off  arith_type="Signed  (2's comp)"  force_bin_pt=on  bin_pt=19  block_type=reinterpret
  tweak_op : xbsIndex_r4/Logical  logical_function=AND  inputs=2  en=off  latency=0  precision=Full  arith_type=Unsigned  n_bits=8  bin_pt=2  align_bp=on  dbl_ovrd=off  block_type=logical
  out : Outport
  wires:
  tweak_op/1 -> Concat/2
  Constant/1 -> tweak_op/2
  bit/1 -> tweak_op/1
  almost_half/1 -> force2/1
  in/1 -> Reinterpret/1, bit/1
  Concat/1 -> force1/1
  Reinterpret/1 -> Concat/1
  force1/1 -> adder/1
  force2/1 -> adder/2
  adder/1 -> out/1

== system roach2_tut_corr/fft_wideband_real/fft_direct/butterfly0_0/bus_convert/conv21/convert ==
  note: (ones_bit & 1) -> round-to-even (ones_bit ^ 1) -> round-to-odd (sign_bit & 1)-> round-to-zero (sign_bit ^ 1) -> round-to-inf (X ~| 1) -> round half down (X | 1) -> round half up
  in : Inport
  Concat : xbsIndex_r4/Concat  num_inputs=2  dbl_ovrd=off  block_type=concat
  Constant : xbsIndex_r4/Constant  const=1  gui_display_data_type=Fixed-point  arith_type=Unsigned  n_bits=1  bin_pt=0  preci_type=Single  exp_width=8  frac_width=24  explicit_period=off  period=1  equ=P=C  opselect=C  inp2=PCIN>>17  opr=+  inp1=P  carry=CIN  dbl_ovrd=off  block_type=constant
  Reinterpret : xbsIndex_r4/Reinterpret  force_arith_type=on  arith_type=Unsigned  force_bin_pt=on  bin_pt=0  block_type=reinterpret
  adder : xbsIndex_r4/AddSub  mode=Addition  use_carryin=off  use_carryout=off  en=off  latency=1  precision=User Defined  arith_type="Signed  (2's comp)"  n_bits=18  bin_pt=17  quantization=Truncate  overflow=Wrap  dbl_ovrd=off  use_behavioral_HDL=off  hw_selection=Fabric  pipelined=on  use_rpm=on  block_type=addsub
  almost_half : xbsIndex_r4/Constant  const=1  gui_display_data_type=Fixed-point  arith_type=Unsigned  n_bits=19  bin_pt=0  preci_type=Single  exp_width=8  frac_width=24  explicit_period=off  period=1  equ=P=C  opselect=C  inp2=PCIN>>17  opr=+  inp1=P  carry=CIN  dbl_ovrd=off  block_type=constant
  bit : xbsIndex_r4/Slice  nbits=1  boolean_output=off  mode=Lower Bit Location + Width  bit1=0  base1=MSB of Input  bit0=1  base0=LSB of Input  dbl_ovrd=off  block_type=slice
  force1 : xbsIndex_r4/Reinterpret  force_arith_type=on  arith_type="Signed  (2's comp)"  force_bin_pt=on  bin_pt=19  block_type=reinterpret
  force2 : xbsIndex_r4/Reinterpret  force_arith_type=off  arith_type="Signed  (2's comp)"  force_bin_pt=on  bin_pt=19  block_type=reinterpret
  tweak_op : xbsIndex_r4/Logical  logical_function=AND  inputs=2  en=off  latency=0  precision=Full  arith_type=Unsigned  n_bits=8  bin_pt=2  align_bp=on  dbl_ovrd=off  block_type=logical
  out : Outport
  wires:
  tweak_op/1 -> Concat/2
  Constant/1 -> tweak_op/2
  bit/1 -> tweak_op/1
  almost_half/1 -> force2/1
  in/1 -> Reinterpret/1, bit/1
  Concat/1 -> force1/1
  Reinterpret/1 -> Concat/1
  force1/1 -> adder/1
  force2/1 -> adder/2
  adder/1 -> out/1

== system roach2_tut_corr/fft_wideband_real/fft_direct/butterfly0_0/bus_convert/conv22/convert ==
  note: (ones_bit & 1) -> round-to-even (ones_bit ^ 1) -> round-to-odd (sign_bit & 1)-> round-to-zero (sign_bit ^ 1) -> round-to-inf (X ~| 1) -> round half down (X | 1) -> round half up
  in : Inport
  Concat : xbsIndex_r4/Concat  num_inputs=2  dbl_ovrd=off  block_type=concat
  Constant : xbsIndex_r4/Constant  const=1  gui_display_data_type=Fixed-point  arith_type=Unsigned  n_bits=1  bin_pt=0  preci_type=Single  exp_width=8  frac_width=24  explicit_period=off  period=1  equ=P=C  opselect=C  inp2=PCIN>>17  opr=+  inp1=P  carry=CIN  dbl_ovrd=off  block_type=constant
  Reinterpret : xbsIndex_r4/Reinterpret  force_arith_type=on  arith_type=Unsigned  force_bin_pt=on  bin_pt=0  block_type=reinterpret
  adder : xbsIndex_r4/AddSub  mode=Addition  use_carryin=off  use_carryout=off  en=off  latency=1  precision=User Defined  arith_type="Signed  (2's comp)"  n_bits=18  bin_pt=17  quantization=Truncate  overflow=Wrap  dbl_ovrd=off  use_behavioral_HDL=off  hw_selection=Fabric  pipelined=on  use_rpm=on  block_type=addsub
  almost_half : xbsIndex_r4/Constant  const=1  gui_display_data_type=Fixed-point  arith_type=Unsigned  n_bits=19  bin_pt=0  preci_type=Single  exp_width=8  frac_width=24  explicit_period=off  period=1  equ=P=C  opselect=C  inp2=PCIN>>17  opr=+  inp1=P  carry=CIN  dbl_ovrd=off  block_type=constant
  bit : xbsIndex_r4/Slice  nbits=1  boolean_output=off  mode=Lower Bit Location + Width  bit1=0  base1=MSB of Input  bit0=1  base0=LSB of Input  dbl_ovrd=off  block_type=slice
  force1 : xbsIndex_r4/Reinterpret  force_arith_type=on  arith_type="Signed  (2's comp)"  force_bin_pt=on  bin_pt=19  block_type=reinterpret
  force2 : xbsIndex_r4/Reinterpret  force_arith_type=off  arith_type="Signed  (2's comp)"  force_bin_pt=on  bin_pt=19  block_type=reinterpret
  tweak_op : xbsIndex_r4/Logical  logical_function=AND  inputs=2  en=off  latency=0  precision=Full  arith_type=Unsigned  n_bits=8  bin_pt=2  align_bp=on  dbl_ovrd=off  block_type=logical
  out : Outport
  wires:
  tweak_op/1 -> Concat/2
  Constant/1 -> tweak_op/2
  bit/1 -> tweak_op/1
  almost_half/1 -> force2/1
  in/1 -> Reinterpret/1, bit/1
  Concat/1 -> force1/1
  Reinterpret/1 -> Concat/1
  force1/1 -> adder/1
  force2/1 -> adder/2
  adder/1 -> out/1

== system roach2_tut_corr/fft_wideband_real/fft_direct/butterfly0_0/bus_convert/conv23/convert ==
  note: (ones_bit & 1) -> round-to-even (ones_bit ^ 1) -> round-to-odd (sign_bit & 1)-> round-to-zero (sign_bit ^ 1) -> round-to-inf (X ~| 1) -> round half down (X | 1) -> round half up
  in : Inport
  Concat : xbsIndex_r4/Concat  num_inputs=2  dbl_ovrd=off  block_type=concat
  Constant : xbsIndex_r4/Constant  const=1  gui_display_data_type=Fixed-point  arith_type=Unsigned  n_bits=1  bin_pt=0  preci_type=Single  exp_width=8  frac_width=24  explicit_period=off  period=1  equ=P=C  opselect=C  inp2=PCIN>>17  opr=+  inp1=P  carry=CIN  dbl_ovrd=off  block_type=constant
  Reinterpret : xbsIndex_r4/Reinterpret  force_arith_type=on  arith_type=Unsigned  force_bin_pt=on  bin_pt=0  block_type=reinterpret
  adder : xbsIndex_r4/AddSub  mode=Addition  use_carryin=off  use_carryout=off  en=off  latency=1  precision=User Defined  arith_type="Signed  (2's comp)"  n_bits=18  bin_pt=17  quantization=Truncate  overflow=Wrap  dbl_ovrd=off  use_behavioral_HDL=off  hw_selection=Fabric  pipelined=on  use_rpm=on  block_type=addsub
  almost_half : xbsIndex_r4/Constant  const=1  gui_display_data_type=Fixed-point  arith_type=Unsigned  n_bits=19  bin_pt=0  preci_type=Single  exp_width=8  frac_width=24  explicit_period=off  period=1  equ=P=C  opselect=C  inp2=PCIN>>17  opr=+  inp1=P  carry=CIN  dbl_ovrd=off  block_type=constant
  bit : xbsIndex_r4/Slice  nbits=1  boolean_output=off  mode=Lower Bit Location + Width  bit1=0  base1=MSB of Input  bit0=1  base0=LSB of Input  dbl_ovrd=off  block_type=slice
  force1 : xbsIndex_r4/Reinterpret  force_arith_type=on  arith_type="Signed  (2's comp)"  force_bin_pt=on  bin_pt=19  block_type=reinterpret
  force2 : xbsIndex_r4/Reinterpret  force_arith_type=off  arith_type="Signed  (2's comp)"  force_bin_pt=on  bin_pt=19  block_type=reinterpret
  tweak_op : xbsIndex_r4/Logical  logical_function=AND  inputs=2  en=off  latency=0  precision=Full  arith_type=Unsigned  n_bits=8  bin_pt=2  align_bp=on  dbl_ovrd=off  block_type=logical
  out : Outport
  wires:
  tweak_op/1 -> Concat/2
  Constant/1 -> tweak_op/2
  bit/1 -> tweak_op/1
  almost_half/1 -> force2/1
  in/1 -> Reinterpret/1, bit/1
  Concat/1 -> force1/1
  Reinterpret/1 -> Concat/1
  force1/1 -> adder/1
  force2/1 -> adder/2
  adder/1 -> out/1

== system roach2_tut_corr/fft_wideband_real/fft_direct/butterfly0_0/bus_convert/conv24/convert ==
  note: (ones_bit & 1) -> round-to-even (ones_bit ^ 1) -> round-to-odd (sign_bit & 1)-> round-to-zero (sign_bit ^ 1) -> round-to-inf (X ~| 1) -> round half down (X | 1) -> round half up
  in : Inport
  Concat : xbsIndex_r4/Concat  num_inputs=2  dbl_ovrd=off  block_type=concat
  Constant : xbsIndex_r4/Constant  const=1  gui_display_data_type=Fixed-point  arith_type=Unsigned  n_bits=1  bin_pt=0  preci_type=Single  exp_width=8  frac_width=24  explicit_period=off  period=1  equ=P=C  opselect=C  inp2=PCIN>>17  opr=+  inp1=P  carry=CIN  dbl_ovrd=off  block_type=constant
  Reinterpret : xbsIndex_r4/Reinterpret  force_arith_type=on  arith_type=Unsigned  force_bin_pt=on  bin_pt=0  block_type=reinterpret
  adder : xbsIndex_r4/AddSub  mode=Addition  use_carryin=off  use_carryout=off  en=off  latency=1  precision=User Defined  arith_type="Signed  (2's comp)"  n_bits=18  bin_pt=17  quantization=Truncate  overflow=Wrap  dbl_ovrd=off  use_behavioral_HDL=off  hw_selection=Fabric  pipelined=on  use_rpm=on  block_type=addsub
  almost_half : xbsIndex_r4/Constant  const=1  gui_display_data_type=Fixed-point  arith_type=Unsigned  n_bits=19  bin_pt=0  preci_type=Single  exp_width=8  frac_width=24  explicit_period=off  period=1  equ=P=C  opselect=C  inp2=PCIN>>17  opr=+  inp1=P  carry=CIN  dbl_ovrd=off  block_type=constant
  bit : xbsIndex_r4/Slice  nbits=1  boolean_output=off  mode=Lower Bit Location + Width  bit1=0  base1=MSB of Input  bit0=1  base0=LSB of Input  dbl_ovrd=off  block_type=slice
  force1 : xbsIndex_r4/Reinterpret  force_arith_type=on  arith_type="Signed  (2's comp)"  force_bin_pt=on  bin_pt=19  block_type=reinterpret
  force2 : xbsIndex_r4/Reinterpret  force_arith_type=off  arith_type="Signed  (2's comp)"  force_bin_pt=on  bin_pt=19  block_type=reinterpret
  tweak_op : xbsIndex_r4/Logical  logical_function=AND  inputs=2  en=off  latency=0  precision=Full  arith_type=Unsigned  n_bits=8  bin_pt=2  align_bp=on  dbl_ovrd=off  block_type=logical
  out : Outport
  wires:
  tweak_op/1 -> Concat/2
  Constant/1 -> tweak_op/2
  bit/1 -> tweak_op/1
  almost_half/1 -> force2/1
  in/1 -> Reinterpret/1, bit/1
  Concat/1 -> force1/1
  Reinterpret/1 -> Concat/1
  force1/1 -> adder/1
  force2/1 -> adder/2
  adder/1 -> out/1

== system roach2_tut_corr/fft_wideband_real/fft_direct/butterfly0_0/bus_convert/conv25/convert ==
  note: (ones_bit & 1) -> round-to-even (ones_bit ^ 1) -> round-to-odd (sign_bit & 1)-> round-to-zero (sign_bit ^ 1) -> round-to-inf (X ~| 1) -> round half down (X | 1) -> round half up
  in : Inport
  Concat : xbsIndex_r4/Concat  num_inputs=2  dbl_ovrd=off  block_type=concat
  Constant : xbsIndex_r4/Constant  const=1  gui_display_data_type=Fixed-point  arith_type=Unsigned  n_bits=1  bin_pt=0  preci_type=Single  exp_width=8  frac_width=24  explicit_period=off  period=1  equ=P=C  opselect=C  inp2=PCIN>>17  opr=+  inp1=P  carry=CIN  dbl_ovrd=off  block_type=constant
  Reinterpret : xbsIndex_r4/Reinterpret  force_arith_type=on  arith_type=Unsigned  force_bin_pt=on  bin_pt=0  block_type=reinterpret
  adder : xbsIndex_r4/AddSub  mode=Addition  use_carryin=off  use_carryout=off  en=off  latency=1  precision=User Defined  arith_type="Signed  (2's comp)"  n_bits=18  bin_pt=17  quantization=Truncate  overflow=Wrap  dbl_ovrd=off  use_behavioral_HDL=off  hw_selection=Fabric  pipelined=on  use_rpm=on  block_type=addsub
  almost_half : xbsIndex_r4/Constant  const=1  gui_display_data_type=Fixed-point  arith_type=Unsigned  n_bits=19  bin_pt=0  preci_type=Single  exp_width=8  frac_width=24  explicit_period=off  period=1  equ=P=C  opselect=C  inp2=PCIN>>17  opr=+  inp1=P  carry=CIN  dbl_ovrd=off  block_type=constant
  bit : xbsIndex_r4/Slice  nbits=1  boolean_output=off  mode=Lower Bit Location + Width  bit1=0  base1=MSB of Input  bit0=1  base0=LSB of Input  dbl_ovrd=off  block_type=slice
  force1 : xbsIndex_r4/Reinterpret  force_arith_type=on  arith_type="Signed  (2's comp)"  force_bin_pt=on  bin_pt=19  block_type=reinterpret
  force2 : xbsIndex_r4/Reinterpret  force_arith_type=off  arith_type="Signed  (2's comp)"  force_bin_pt=on  bin_pt=19  block_type=reinterpret
  tweak_op : xbsIndex_r4/Logical  logical_function=AND  inputs=2  en=off  latency=0  precision=Full  arith_type=Unsigned  n_bits=8  bin_pt=2  align_bp=on  dbl_ovrd=off  block_type=logical
  out : Outport
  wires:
  tweak_op/1 -> Concat/2
  Constant/1 -> tweak_op/2
  bit/1 -> tweak_op/1
  almost_half/1 -> force2/1
  in/1 -> Reinterpret/1, bit/1
  Concat/1 -> force1/1
  Reinterpret/1 -> Concat/1
  force1/1 -> adder/1
  force2/1 -> adder/2
  adder/1 -> out/1

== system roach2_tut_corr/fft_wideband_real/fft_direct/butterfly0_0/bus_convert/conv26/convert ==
  note: (ones_bit & 1) -> round-to-even (ones_bit ^ 1) -> round-to-odd (sign_bit & 1)-> round-to-zero (sign_bit ^ 1) -> round-to-inf (X ~| 1) -> round half down (X | 1) -> round half up
  in : Inport
  Concat : xbsIndex_r4/Concat  num_inputs=2  dbl_ovrd=off  block_type=concat
  Constant : xbsIndex_r4/Constant  const=1  gui_display_data_type=Fixed-point  arith_type=Unsigned  n_bits=1  bin_pt=0  preci_type=Single  exp_width=8  frac_width=24  explicit_period=off  period=1  equ=P=C  opselect=C  inp2=PCIN>>17  opr=+  inp1=P  carry=CIN  dbl_ovrd=off  block_type=constant
  Reinterpret : xbsIndex_r4/Reinterpret  force_arith_type=on  arith_type=Unsigned  force_bin_pt=on  bin_pt=0  block_type=reinterpret
  adder : xbsIndex_r4/AddSub  mode=Addition  use_carryin=off  use_carryout=off  en=off  latency=1  precision=User Defined  arith_type="Signed  (2's comp)"  n_bits=18  bin_pt=17  quantization=Truncate  overflow=Wrap  dbl_ovrd=off  use_behavioral_HDL=off  hw_selection=Fabric  pipelined=on  use_rpm=on  block_type=addsub
  almost_half : xbsIndex_r4/Constant  const=1  gui_display_data_type=Fixed-point  arith_type=Unsigned  n_bits=19  bin_pt=0  preci_type=Single  exp_width=8  frac_width=24  explicit_period=off  period=1  equ=P=C  opselect=C  inp2=PCIN>>17  opr=+  inp1=P  carry=CIN  dbl_ovrd=off  block_type=constant
  bit : xbsIndex_r4/Slice  nbits=1  boolean_output=off  mode=Lower Bit Location + Width  bit1=0  base1=MSB of Input  bit0=1  base0=LSB of Input  dbl_ovrd=off  block_type=slice
  force1 : xbsIndex_r4/Reinterpret  force_arith_type=on  arith_type="Signed  (2's comp)"  force_bin_pt=on  bin_pt=19  block_type=reinterpret
  force2 : xbsIndex_r4/Reinterpret  force_arith_type=off  arith_type="Signed  (2's comp)"  force_bin_pt=on  bin_pt=19  block_type=reinterpret
  tweak_op : xbsIndex_r4/Logical  logical_function=AND  inputs=2  en=off  latency=0  precision=Full  arith_type=Unsigned  n_bits=8  bin_pt=2  align_bp=on  dbl_ovrd=off  block_type=logical
  out : Outport
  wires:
  tweak_op/1 -> Concat/2
  Constant/1 -> tweak_op/2
  bit/1 -> tweak_op/1
  almost_half/1 -> force2/1
  in/1 -> Reinterpret/1, bit/1
  Concat/1 -> force1/1
  Reinterpret/1 -> Concat/1
  force1/1 -> adder/1
  force2/1 -> adder/2
  adder/1 -> out/1

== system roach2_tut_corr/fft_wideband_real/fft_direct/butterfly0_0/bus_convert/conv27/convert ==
  note: (ones_bit & 1) -> round-to-even (ones_bit ^ 1) -> round-to-odd (sign_bit & 1)-> round-to-zero (sign_bit ^ 1) -> round-to-inf (X ~| 1) -> round half down (X | 1) -> round half up
  in : Inport
  Concat : xbsIndex_r4/Concat  num_inputs=2  dbl_ovrd=off  block_type=concat
  Constant : xbsIndex_r4/Constant  const=1  gui_display_data_type=Fixed-point  arith_type=Unsigned  n_bits=1  bin_pt=0  preci_type=Single  exp_width=8  frac_width=24  explicit_period=off  period=1  equ=P=C  opselect=C  inp2=PCIN>>17  opr=+  inp1=P  carry=CIN  dbl_ovrd=off  block_type=constant
  Reinterpret : xbsIndex_r4/Reinterpret  force_arith_type=on  arith_type=Unsigned  force_bin_pt=on  bin_pt=0  block_type=reinterpret
  adder : xbsIndex_r4/AddSub  mode=Addition  use_carryin=off  use_carryout=off  en=off  latency=1  precision=User Defined  arith_type="Signed  (2's comp)"  n_bits=18  bin_pt=17  quantization=Truncate  overflow=Wrap  dbl_ovrd=off  use_behavioral_HDL=off  hw_selection=Fabric  pipelined=on  use_rpm=on  block_type=addsub
  almost_half : xbsIndex_r4/Constant  const=1  gui_display_data_type=Fixed-point  arith_type=Unsigned  n_bits=19  bin_pt=0  preci_type=Single  exp_width=8  frac_width=24  explicit_period=off  period=1  equ=P=C  opselect=C  inp2=PCIN>>17  opr=+  inp1=P  carry=CIN  dbl_ovrd=off  block_type=constant
  bit : xbsIndex_r4/Slice  nbits=1  boolean_output=off  mode=Lower Bit Location + Width  bit1=0  base1=MSB of Input  bit0=1  base0=LSB of Input  dbl_ovrd=off  block_type=slice
  force1 : xbsIndex_r4/Reinterpret  force_arith_type=on  arith_type="Signed  (2's comp)"  force_bin_pt=on  bin_pt=19  block_type=reinterpret
  force2 : xbsIndex_r4/Reinterpret  force_arith_type=off  arith_type="Signed  (2's comp)"  force_bin_pt=on  bin_pt=19  block_type=reinterpret
  tweak_op : xbsIndex_r4/Logical  logical_function=AND  inputs=2  en=off  latency=0  precision=Full  arith_type=Unsigned  n_bits=8  bin_pt=2  align_bp=on  dbl_ovrd=off  block_type=logical
  out : Outport
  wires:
  tweak_op/1 -> Concat/2
  Constant/1 -> tweak_op/2
  bit/1 -> tweak_op/1
  almost_half/1 -> force2/1
  in/1 -> Reinterpret/1, bit/1
  Concat/1 -> force1/1
  Reinterpret/1 -> Concat/1
  force1/1 -> adder/1
  force2/1 -> adder/2
  adder/1 -> out/1

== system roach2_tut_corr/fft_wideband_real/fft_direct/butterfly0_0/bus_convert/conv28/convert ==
  note: (ones_bit & 1) -> round-to-even (ones_bit ^ 1) -> round-to-odd (sign_bit & 1)-> round-to-zero (sign_bit ^ 1) -> round-to-inf (X ~| 1) -> round half down (X | 1) -> round half up
  in : Inport
  Concat : xbsIndex_r4/Concat  num_inputs=2  dbl_ovrd=off  block_type=concat
  Constant : xbsIndex_r4/Constant  const=1  gui_display_data_type=Fixed-point  arith_type=Unsigned  n_bits=1  bin_pt=0  preci_type=Single  exp_width=8  frac_width=24  explicit_period=off  period=1  equ=P=C  opselect=C  inp2=PCIN>>17  opr=+  inp1=P  carry=CIN  dbl_ovrd=off  block_type=constant
  Reinterpret : xbsIndex_r4/Reinterpret  force_arith_type=on  arith_type=Unsigned  force_bin_pt=on  bin_pt=0  block_type=reinterpret
  adder : xbsIndex_r4/AddSub  mode=Addition  use_carryin=off  use_carryout=off  en=off  latency=1  precision=User Defined  arith_type="Signed  (2's comp)"  n_bits=18  bin_pt=17  quantization=Truncate  overflow=Wrap  dbl_ovrd=off  use_behavioral_HDL=off  hw_selection=Fabric  pipelined=on  use_rpm=on  block_type=addsub
  almost_half : xbsIndex_r4/Constant  const=1  gui_display_data_type=Fixed-point  arith_type=Unsigned  n_bits=19  bin_pt=0  preci_type=Single  exp_width=8  frac_width=24  explicit_period=off  period=1  equ=P=C  opselect=C  inp2=PCIN>>17  opr=+  inp1=P  carry=CIN  dbl_ovrd=off  block_type=constant
  bit : xbsIndex_r4/Slice  nbits=1  boolean_output=off  mode=Lower Bit Location + Width  bit1=0  base1=MSB of Input  bit0=1  base0=LSB of Input  dbl_ovrd=off  block_type=slice
  force1 : xbsIndex_r4/Reinterpret  force_arith_type=on  arith_type="Signed  (2's comp)"  force_bin_pt=on  bin_pt=19  block_type=reinterpret
  force2 : xbsIndex_r4/Reinterpret  force_arith_type=off  arith_type="Signed  (2's comp)"  force_bin_pt=on  bin_pt=19  block_type=reinterpret
  tweak_op : xbsIndex_r4/Logical  logical_function=AND  inputs=2  en=off  latency=0  precision=Full  arith_type=Unsigned  n_bits=8  bin_pt=2  align_bp=on  dbl_ovrd=off  block_type=logical
  out : Outport
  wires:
  tweak_op/1 -> Concat/2
  Constant/1 -> tweak_op/2
  bit/1 -> tweak_op/1
  almost_half/1 -> force2/1
  in/1 -> Reinterpret/1, bit/1
  Concat/1 -> force1/1
  Reinterpret/1 -> Concat/1
  force1/1 -> adder/1
  force2/1 -> adder/2
  adder/1 -> out/1
